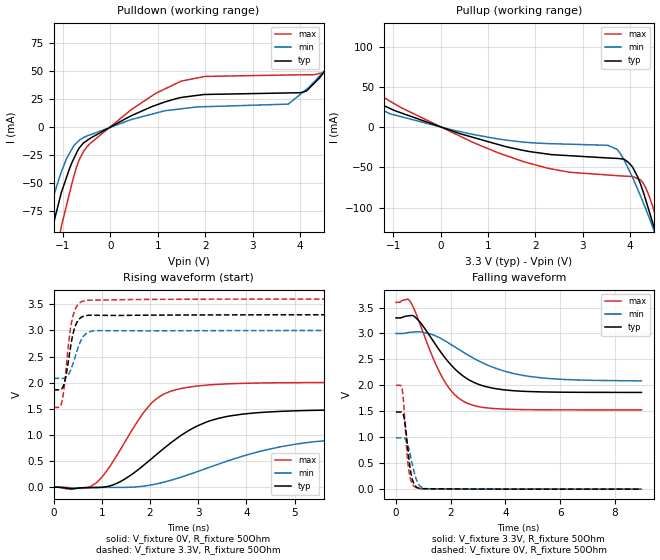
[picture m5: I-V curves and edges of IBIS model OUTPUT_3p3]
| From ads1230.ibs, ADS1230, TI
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|   Output OUTPUT 3V Model
[Model] OUTPUT_3p3
Model_type Output
|Signal _DRDY_DOUT(16) pin
Polarity   Non-Inverting
Enable   Active-Low
Vmeas = 1.65
Vref = 1.65
Cref = 15pF
Rref = 50
|   typ   min   max
|   (nom PVT)   (Fast PVT)   (slow PVT)
|Average
C_comp   4.348e-12   3.952e-12   4.513e-12
|ON state : BUFFER OUTPUT TURNED HIGH
|C_comp   4.089e-12   3.912e-12   4.348e-12
|OFF state: BUFFER in HIGH IMPEDANCE for IOs and 3-state,
|This is BUFFER in LOW state for OUTPUT only type
|C_comp   4.182e-12   3.991e-12   4.936e-12
| Where   nom PVT is  Nominal Process, 3.3V, 25C
|   Fast PVT is Strong Process, 3.6V, -40C
|   Slow PVT is Weak Process, 3.0V, 85C
[Voltage Range]   3.3   3   3.6
|Ambient Temperature   25   85   -40
|Junction Temperature
[Temperature Range]   25   85   -40
[Pullup Reference]   3.3   3   3.6
[Pulldown Reference]   0   0   0
[Power Clamp Reference]   3.3   3   3.6
[GND Clamp Reference]   0   0   0
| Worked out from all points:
|   slope of the pulldown table from 0 to 0.495 V, typ, clamps not added: 44.4 ohm
|   slope of the pullup table from 0 to 0.495 V, typ, clamps not added: 49.8 ohm
|   falling waveform, V_fixture 3.3V, R_fixture 50Ohm: 20-80 % time 1.37ns typ, 2.08ns min, 1.07ns max; typ from 3.3 V to 1.86 V
|   rising waveform, V_fixture 0V, R_fixture 50Ohm: 20-80 % time 1.33ns typ, 2.13ns min, 857ps max; typ from 0 V to 1.49 V
|   rising waveform, V_fixture 3.3V, R_fixture 50Ohm: 20-80 % time 163ps typ, 206ps min, 156ps max; typ from 1.86 V to 3.3 V
|   falling waveform, V_fixture 0V, R_fixture 50Ohm: 20-80 % time 201ps typ, 274ps min, 171ps max; typ from 1.49 V to 0 V
[Pulldown]
|   Voltage   I(typ)   I(min)   I(max)
-3.3V     -563.8mA   -410.1mA   -812.5mA
-1.554V   -160mA     -113.4mA   -230.7mA
-1.363V   -118.8mA   -84.64mA   -170.7mA
-1.183V   -83.23mA   -59.38mA   -120.3mA
-1.036V   -58.47mA   -39.99mA   -88.86mA
-715.2mV  -23.1mA    -14.12mA   -35.48mA
-492mV    -11.87mA   -7.755mA   -17.48mA
1.492V    26.42mA    16.32mA    40.91mA
3.753V    30.45mA    20.48mA    46.46mA
4.508V    49.05mA    49.5mA     48.74mA
5.495V    103.7mA    91.79mA    119.6mA
6.6V      156.4mA    131.3mA    192.8mA
[Pullup]
|   Voltage   I(typ)   I(min)   I(max)
-3.3V     124.1mA    101.4mA    158.5mA
-2.576V   93.35mA    75.84mA    120.1mA
-1.572V   41.65mA    34.03mA    52.46mA
-970.2mV  20.59mA    15.1mA     28.98mA
1.758V    -29.1mA    -18.69mA   -43.05mA
3.723V    -38.88mA   -27.5mA    -60.34mA
4.043V    -48.86mA   -61.29mA   -61.38mA
4.224V    -71.41mA   -86.16mA   -65.79mA
4.483V    -120mA     -125.1mA   -99.53mA
4.552V    -134.1mA   -135.8mA   -112.9mA
4.623V    -149.2mA   -146.9mA   -129.3mA
6.6V      -606.2mA   -488.2mA   -776.3mA
[Ramp]
R_load = 50
|   typ   min   max
dV/dt_r   0.892575/1.3207e-09   0.589759/2.12513e-09   1.20285/8.57115e-10
dV/dt_f   0.861501/1.37213e-09   0.547859/2.07387e-09   1.24372/1.07195e-09
[Falling Waveform]
V_fixture = 3.3V
V_fixture_min = 3V
V_fixture_max = 3.6V
R_fixture = 50Ohm
C_fixture = 0F
|   Time   V(typ)   V(min)   V(max)
0s        3.3V       3V         3.6V
525ps     3.344V     3.023V     3.612V
875ps     3.219V     3.033V     3.187V
1.35ns    2.862V     2.974V     2.535V
1.725ns   2.579V     2.879V     2.123V
2.125ns   2.331V     2.75V      1.833V
2.625ns   2.12V      2.587V     1.652V
3.525ns   1.947V     2.353V     1.556V
4.825ns   1.882V     2.177V     1.532V
8.975ns   1.864V     2.087V     1.527V
[Rising Waveform]
V_fixture = 0V
V_fixture_min = 0V
V_fixture_max = 0V
R_fixture = 50Ohm
C_fixture = 0F
|   Time   V(typ)   V(min)   V(max)
0s        1.028nV    1.153nV    865.2pV
350ps     -25.63mV   -9.442mV   -36.82mV
875ps     -5.717mV   -4.63mV    76.82mV
1.375ns   102.3mV    -3.17mV    702.4mV
2ns       520.3mV    39.56mV    1.578V
2.25ns    714.3mV    88.58mV    1.764V
2.6ns     963.1mV    180.1mV    1.879V
3.575ns   1.35V      491.5mV    1.977V
5.175ns   1.466V     843.9mV    2.002V
8.975ns   1.488V     982.9mV    2.005V
[Rising Waveform]
V_fixture = 3.3V
V_fixture_min = 3V
V_fixture_max = 3.6V
R_fixture = 50Ohm
C_fixture = 0F
|   Time   V(typ)   V(min)   V(max)
0s        1.864V     2.084V     1.527V
125ps     1.863V     2.084V     1.535V
175ps     1.887V     2.082V     1.635V
250ps     2.091V     2.098V     2.166V
325ps     2.514V     2.182V     2.857V
400ps     2.92V      2.351V     3.265V
500ps     3.179V     2.649V     3.487V
650ps     3.28V      2.917V     3.569V
975ps     3.29V      2.996V     3.581V
8.975ns   3.3V       3V         3.6V
[Falling Waveform]
|Gnd
V_fixture = 0V
V_fixture_min = 0V
V_fixture_max = 0V
R_fixture = 50Ohm
C_fixture = 0F
|   Time   V(typ)   V(min)   V(max)
0s        1.486V     989mV      2.001V
225ps     1.475V     990.2mV    1.927V
275ps     1.422V     987.7mV    1.699V
325ps     1.285V     972.9mV    1.314V
400ps     945.9mV    901.3mV    713.9mV
475ps     578.1mV    764.6mV    340.6mV
600ps     184.2mV    471.2mV    99.79mV
750ps     39.32mV    177.3mV    24.15mV
1.225ns   7.173mV    7.017mV    7.784mV
8.975ns   220uV      315.4uV    78.71uV
